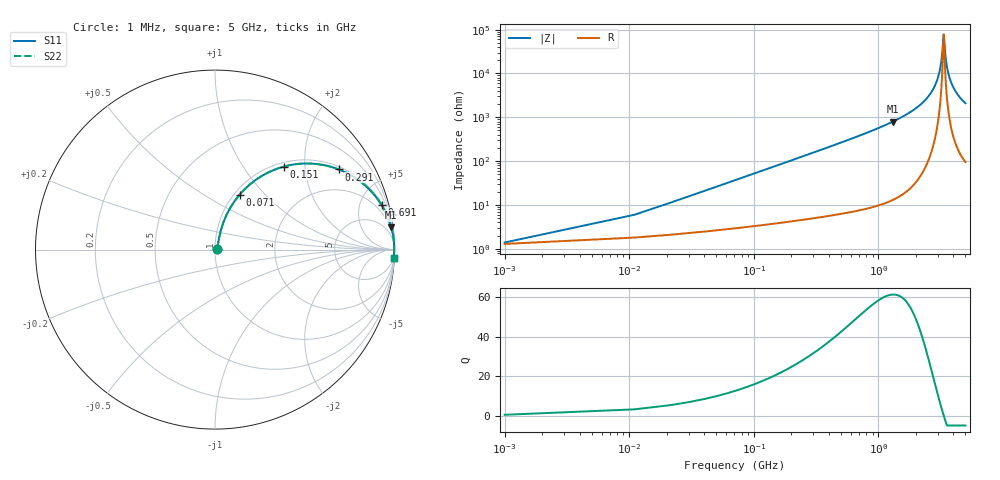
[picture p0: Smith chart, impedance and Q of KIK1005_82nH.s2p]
!version-3
!date-01.2023
!Series
# MHz S RI R 50
!Freq ReS11 ImS11 ReS21 ImS21 ReS12 ImS12 ReS22 ImS22
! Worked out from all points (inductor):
!   501 points, 1 MHz to 5 GHz, reference 50 ohm
!   read as one part in series: L = 82 nH near 21 MHz
!   highest Q = 61.3 at 1.301 GHz (marker M1), where L = 96.6 nH
!   self-resonance near 3.341 GHz
!   S11 on the Smith chart (normalised r, x): 1 MHz: 1.03, +0.01; 71 MHz: 1.06, +0.73; 151 MHz: 1.08, +1.56; 291 MHz: 1.10, +3.02; 691 MHz: 1.15, +7.44; 5 GHz: 3, -42
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1  0.0127 0.00502  0.9873 -0.00502  0.9873 -0.00502  0.0127 0.00502
31  0.0457 0.149  0.9543 -0.149  0.9543 -0.149  0.0457 0.149
51  0.0856 0.2341  0.9144 -0.2341  0.9144 -0.2341  0.0856 0.2341
71  0.1374 0.3067  0.8626 -0.3067  0.8626 -0.3067  0.1374 0.3067
151  0.384 0.4627  0.616 -0.4627  0.616 -0.4627  0.384 0.4627
291  0.6899 0.4467  0.3101 -0.4467  0.3101 -0.4467  0.6899 0.4467
451  0.8424 0.352  0.1576 -0.352  0.1576 -0.352  0.8424 0.352
691  0.9283 0.2482  0.0717 -0.2482  0.0717 -0.2482  0.9283 0.2482
841  0.9519 0.205  0.0481 -0.205  0.0481 -0.205  0.9519 0.205
1301  0.9822 0.1241  0.0178 -0.1241  0.0178 -0.1241  0.9822 0.1241
1671  0.991 0.0863  0.00902 -0.0863  0.00902 -0.0863  0.991 0.0863
2501  0.9977 0.0342  0.00232 -0.0342  0.00232 -0.0342  0.9977 0.0342
2851  0.9985 0.0187  0.00152 -0.0187  0.00152 -0.0187  0.9985 0.0187
3081  0.9987 0.00966  0.0013 -0.00966  0.0013 -0.00966  0.9987 0.00966
3221  0.9987 0.00451  0.00127 -0.00451  0.00127 -0.00451  0.9987 0.00451
3341  0.9987 0.000283  0.00128 -0.000283  0.00128 -0.000283  0.9987 0.000283
3371  0.9987 -0.00075  0.00129 0.00075  0.00129 0.00075  0.9987 -0.00075
3481  0.9987 -0.00446  0.00135 0.00446  0.00135 0.00446  0.9987 -0.00446
3621  0.9985 -0.00902  0.00146 0.00902  0.00146 0.00902  0.9985 -0.00902
3851  0.9983 -0.0162  0.00174 0.0162  0.00174 0.0162  0.9983 -0.0162
4171  0.9977 -0.0255  0.0023 0.0255  0.0023 0.0255  0.9977 -0.0255
5000  0.9956 -0.0474  0.00442 0.0474  0.00442 0.0474  0.9956 -0.0474
